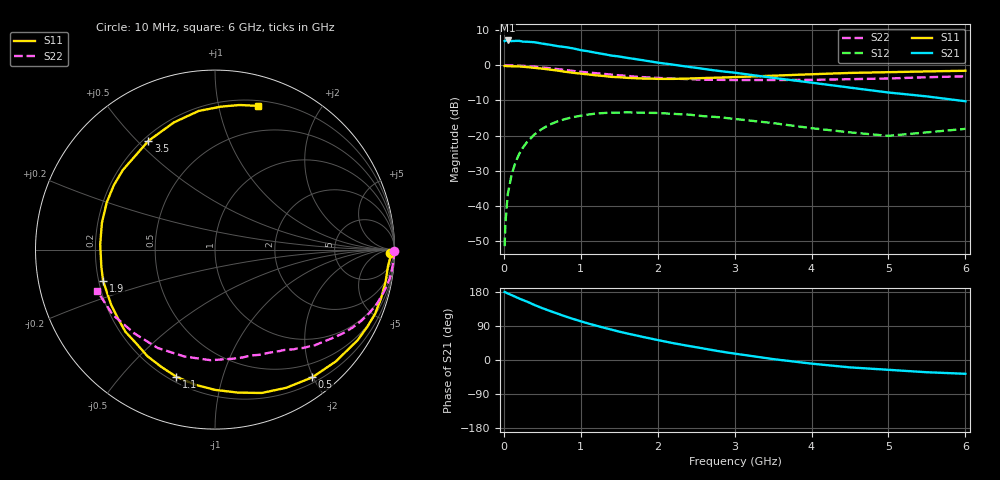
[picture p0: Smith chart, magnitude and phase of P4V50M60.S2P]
! SIEMENS Small Signal Semiconductors
! BFP182
! Si NPN RF Bipolar Junction Transistor in SOT143
! VCE = 0.5 V  IC = 0.6 mA
! Common Emitter S-Parameters:  March  1996
# GHz  S  MA  R  50
!  f  S11  S21  S12  S22
! GHz  MAG  ANG  MAG  ANG  MAG  ANG  MAG  ANG
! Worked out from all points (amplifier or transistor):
!   36 points, 10 MHz to 6 GHz, reference 50 ohm
!   highest |S21| = 7.0 dB at 50 MHz (marker M1)
!   |S21| within 3 dB of that: start of sweep to 1.074 GHz
!   unconditionally stable (mu >= 1): 2.6 GHz to end of sweep
!   at 250 MHz: K = 0.11, MSG = 15.0 dB, |S12| = -23.3 dB
!   at 1.4 GHz: K = 0.57, MSG = 8.1 dB, |S12| = -13.5 dB
!   at 6 GHz: K = 1.66, MAG = -0.8 dB, |S12| = -18.1 dB
!   S11 on the Smith chart (normalised r, x): 10 MHz: 51, -40; 500 MHz: 0.28, -1.99; 1.1 GHz: 0.23, -0.71; 1.9 GHz: 0.22, -0.13; 3.5 GHz: 0.22, +0.54; 6 GHz: 0.25, +1.31
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0.01  0.9759 -1.1  2.202 179.5  0.0027 84.3  0.9984 -0.4
0.02  0.9784 -2.4  2.23 178.9  0.0056 90.4  0.9934 -0.9
0.05  0.9682 -5.6  2.248 175.6  0.0145 87.2  0.9978 -2.3
0.1  0.9672 -10.6  2.201 171.3  0.0278 82.1  0.9942 -4.7
0.2  0.961 -21.9  2.217 162.2  0.0552 75.4  0.9867 -9.4
0.4  0.9172 -42.8  2.122 145.0  0.1046 61.7  0.9523 -18.3
0.5  0.8945 -52.7  2.027 136.8  0.1255 55.1  0.9292 -22.4
0.6  0.8663 -62.7  1.954 129.4  0.144 49.1  0.9062 -26.0
0.8  0.8063 -81.1  1.811 115.0  0.1724 38.0  0.8562 -32.7
0.9  0.7812 -90.1  1.733 108.4  0.1836 32.9  0.8301 -35.7
1.1  0.7398 -107.1  1.575 96.1  0.1996 23.8  0.7877 -41.0
1.3  0.7031 -122.4  1.437 85.3  0.2098 15.6  0.7527 -45.8
1.5  0.6773 -137.5  1.33 74.9  0.2124 8.6  0.7186 -49.9
1.9  0.6474 -164.4  1.134 57.0  0.2108 -3.1  0.6689 -57.8
2.2  0.6402 177.4  1.019 44.5  0.2041 -10.1  0.6457 -63.3
2.8  0.668 147.7  0.828 23.0  0.1829 -21.4  0.6203 -75.5
3.5  0.7102 121.5  0.662 2.4  0.1509 -28.5  0.6168 -92.2
4  0.7447 107.9  0.566 -9.6  0.1278 -28.6  0.6195 -105.9
4.5  0.7778 96.7  0.481 -19.5  0.1114 -25.4  0.6342 -120.1
5  0.797 87.7  0.41 -25.9  0.0995 -14.1  0.6481 -133.9
5.5  0.8171 80.4  0.361 -32.3  0.1115 -5.8  0.676 -147.7
6  0.8353 73.5  0.308 -36.4  0.125 -2.0  0.6955 -160.7
